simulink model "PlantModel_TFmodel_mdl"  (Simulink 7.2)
settings: Solver=ode45  StartTime=0.0  StopTime=10  RelTol=1e-3
InitFcn:
  | s = tf('s');
  | G_plant = (101*s + 808)/(s^3 + 6*s^2 + 109*s + 404);
  | Gd_plant = tf(c2d(G_plant,Ts,'zoh'))
  | [B_plant,A_plant] = tfdata(Gd_plant,'v');
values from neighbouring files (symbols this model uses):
  Ts = 0.01    [Esercitazione03.m]
undefined symbols (not defined in the file or in its folder): A_plant, polyval
libraries: cstblocks x2, simulink x1

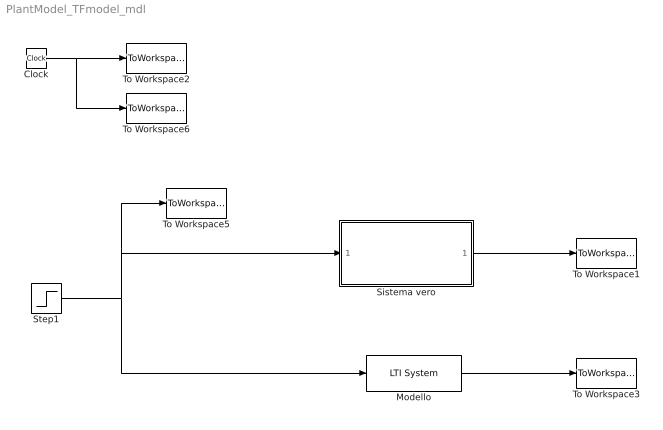
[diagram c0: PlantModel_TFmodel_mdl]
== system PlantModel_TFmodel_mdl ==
  Clock : Clock
  Modello : cstblocks/LTI System  SystemSampleTime=-1  sys=Gz  IC=[]
  Sistema vero : Subsystem
  Step1 : Step  Time=2  SampleTime=0
  To Workspace1 : ToWorkspace  VariableName=y  SampleTime=Ts  SaveFormat=Array
  To Workspace2 : ToWorkspace  VariableName=time  SampleTime=-1  SaveFormat=Array
  To Workspace3 : ToWorkspace  VariableName=ym  SampleTime=Ts  SaveFormat=Array
  To Workspace5 : ToWorkspace  VariableName=u  SampleTime=-1  SaveFormat=Array
  To Workspace6 : ToWorkspace  VariableName=timed  SampleTime=Ts  SaveFormat=Array
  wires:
  Modello/1 -> To Workspace3/1
  Step1/1 -> To Workspace5/1, Sistema vero/1(u), Modello/1
  Sistema vero/1(y) -> To Workspace1/1
  Clock/1 -> To Workspace2/1, To Workspace6/1

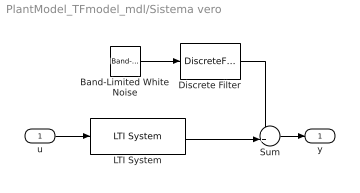
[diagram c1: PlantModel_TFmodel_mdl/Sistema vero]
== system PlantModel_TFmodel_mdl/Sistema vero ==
  u : Inport
  Band-Limited White Noise : simulink/Sources/Band-Limited White Noise  SystemSampleTime=-1  Cov=0.0001  Ts=Ts  seed=[23341]
  Discrete Filter : DiscreteFilter  Numerator=polyval(A_plant,1)*[1]  Denominator=A_plant  SampleTime=Ts
  LTI System : cstblocks/LTI System  SystemSampleTime=-1  sys=Gd_plant  IC=[]
  Sum : Sum  Inputs=++|  OutDataType=sfix(16)  OutScaling=2^0
  y : Outport
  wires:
  LTI System/1 -> Sum/2
  u/1 -> LTI System/1
  Sum/1 -> y/1
  Band-Limited White Noise/1 -> Discrete Filter/1
  Discrete Filter/1 -> Sum/1
